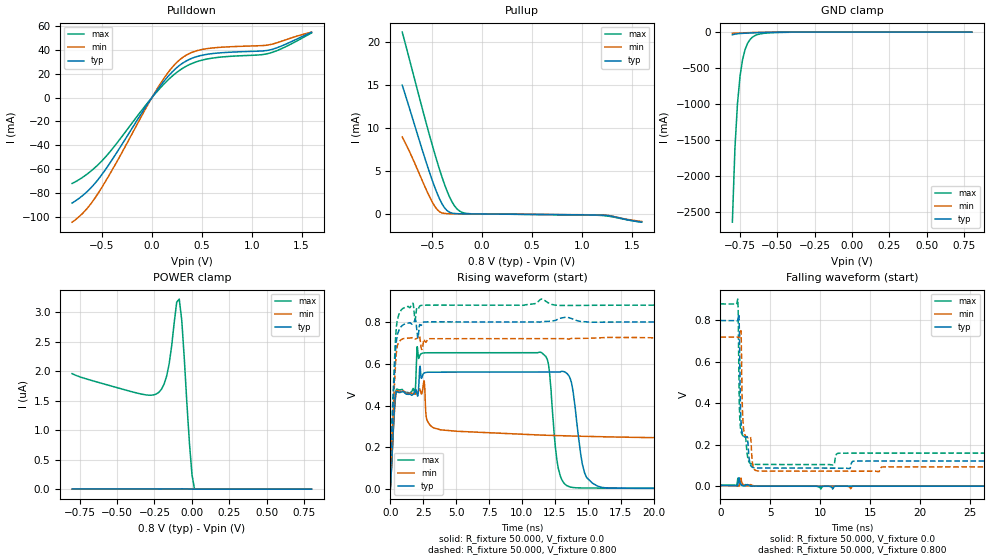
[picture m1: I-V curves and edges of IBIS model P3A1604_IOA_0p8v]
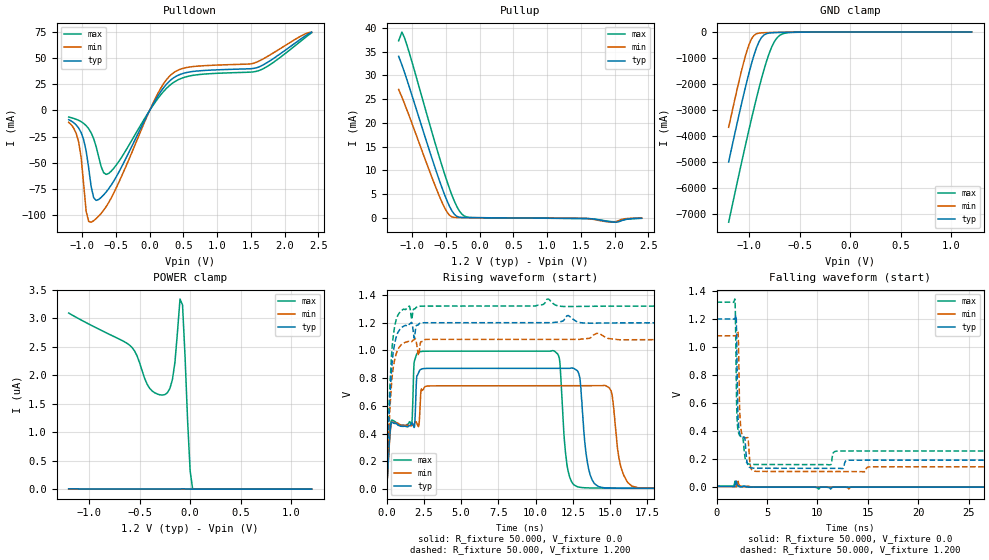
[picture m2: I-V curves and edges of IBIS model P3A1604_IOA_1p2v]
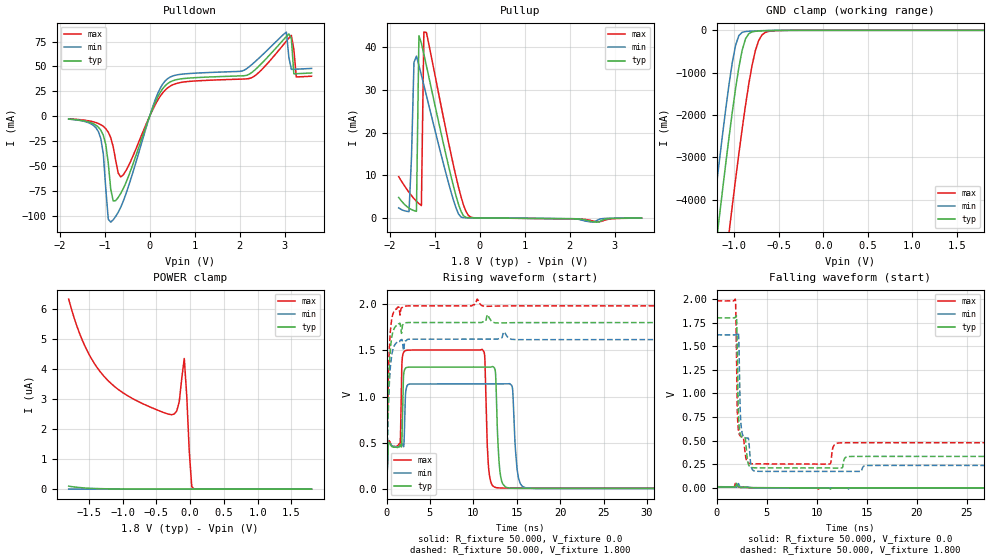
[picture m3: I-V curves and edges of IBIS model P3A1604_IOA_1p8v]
| NXP Semiconductors
| IBIS Model for P3A1604_WLCSP
| BIDIRECTIONAL VOLTAGE LEVEL TRANSLATOR WITH AUTO DIRECTION
| IBIS file created by T2B Version 21.1.4.11121.319246   004
| Cadence Design Systems, Inc. 2011
[IBIS ver] 5.0
[File name] p3a1604_wlcsp.ibs
[File Rev]  1.0
[Date]   July 30, 2024
[Source] NXP
[Notes]   The voltage level for A ports and B ports are
   different,for A side port, the voltage is 0.8v, 1.2V and 1.8V,
   for B side port, the voltage is 1.8v and 3.3V. In
   the model file, the model only contain the node voltage in
   the corresponding range.
   - Pin Description:
   - A1,B1,A2,B2,A3,B3,A4,B4 are the I/O pins.
   - VCCA Supply related to A pin
   - VCCB Supply related to B pin
   - OE is the Enable pin
   - All IO rising/falling waveforms has been verified on Cload=50pF in ADS.
   - IBIS SYNTAX CANNOT DESCRIBE THE CHARACTERISTICS OF
   ANY OUTPUT STRUCTURES THAT DYNAMICALLY CHANGES THE
   IMPEDANCES DURING THE TRANSITION. THIS DEVICE USES SIMILAR
   OUTPUT STRUCTURE AND THEREFORE THE SIMULATION RESULTS
   MAY NOT BE ACCURATE.
[Disclaimer]
NXP Semiconductors warrants and represents that the
IBIS model identified herein is owned by NXP Semiconductors.
The model provided is not warranted as fully representing
all of the operating characteristics and specifications of
the semiconductor products to which the model relates. Moreover,
unless there is a signed, written agreement to the contrary,
this IBIS model is furnished on an "as is" basis without
support or warranty of any kind, either expressed or implied,
regarding the use thereof, and NXP specifically disclaims
all implied warranties of merchantability and fitness of the
model for any purpose. NXP does not assume any liability arising
out of the application or use of this IBIS model including
infringement of patents and copyrights, nor does NXP convey
any license under its patents and copyrights or the rights of
others. NXP provides IBIS models as a service to our customers.
You and your company shall not distribute, convey, sell,
or give these models to anyone else without receiving prior
written permission from NXP Semiconductors.
NXP reserves the right to make changes
without notice to these IBIS models to improve reliability and gain.
This IBIS model is a property of NXP Semiconductors.
|   Component P3A1604
[Component] P3A1604
[Manufacturer] NXP
[Package]
| variable   typ   min   max
R_pkg   19.428m   5.881m   59.711m
L_pkg   1.154nH   1.074nH   1.308nH
C_pkg   0.159pF   0.155pF   0.163pF
[Pin]  signal_name   model_name   R_pin   L_pin   C_pin
B1   B1   P3A1604_IOB
VCCB   VCCB   Power
A1   A1   P3A1604_IOA
B2   B2   P3A1604_IOB
VCCA   VCCA   Power
A2   A2   P3A1604_IOA
B3   B3   P3A1604_IOB
OE   OE   P3A1604_OE
A3   A3   P3A1604_IOA
B4   B4   P3A1604_IOB
GND   GND   GND
A4   A4   P3A1604_IOA
| Model P3A1604_IOB
[Model Selector] 		P3A1604_IOB
P3A1604_IOB_1p8v 		1.8V VCCB supply
P3A1604_IOB_3p3v 		3.3V VCCB supply
| Model P3A1604_IOA
[Model Selector] 		P3A1604_IOA
P3A1604_IOA_0p8v   0.8V VCCA supply
P3A1604_IOA_1p2v 		1.2V VCCA supply
P3A1604_IOA_1p8v 		1.8V VCCA supply
| Model P3A1604_OE
[Model Selector] 		P3A1604_OE
P3A1604_OE_0p8v 		0.8V VCCA supply
P3A1604_OE_1p2v 		1.2V VCCA supply
P3A1604_OE_1p8v 		1.8V VCCA supply
| Models and submodels in the file (8): P3A1604_IOA_0p8v (I/O), P3A1604_IOA_1p2v (I/O), P3A1604_IOA_1p8v (I/O), P3A1604_OE_0p8v (Input), P3A1604_OE_1p2v (Input), P3A1604_OE_1p8v (Input), P3A1604_IOB_1p8v (I/O), P3A1604_IOB_3p3v (I/O)
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|   Model P3A1604_IOA_0p8v
[Model] P3A1604_IOA_0p8v
Model_type I/O
Polarity   Non-Inverting
Enable   Active-High
Vinl =  0.383V
Vinh =  0.407V
C_comp   6.7pF   6.3pF   7.44pF
[Model Spec]
Vinh   0.407V   0.327V   0.497V
Vinl   0.383V   0.309V   0.459V
[Temperature Range]   27.000   -40.000   125
[Voltage Range]   0.800V   0.720V   0.880V
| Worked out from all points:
|   slope of the pulldown table from 0 to 0.12 V, typ, clamps not added: 8.82 ohm
|   slope of the pullup table from 0 to 0.12 V, typ, clamps not added: 10 kohm
|   GND clamp passes 1 mA (typ) near -0.47 V on its own axis
|   rising waveform, R_fixture 50.000, V_fixture 0.800: 20-80 % time 291ps typ, 284ps min, 299ps max; typ from 0.12 V to 0.8 V
|   falling waveform, R_fixture 50.000, V_fixture 0.800: 20-80 % time 272ps typ, 940ps min, 160ps max; typ from 0.8 V to 0.121 V
[Pulldown]
|Voltage   I(typ)   I(min)   I(max)
-800mV    -88.25mA   -104.3mA   -71.84mA
-675mV    -80.6mA    -95.18mA   -65.59mA
-550mV    -69.67mA   -81.51mA   -57mA
-400mV    -52.1mA    -60.81mA   -43.27mA
50mV      5.924mA    7.002mA    4.898mA
175mV     19.01mA    22.42mA    15.82mA
300mV     28.37mA    33.08mA    24.1mA
400mV     32.87mA    37.8mA     28.51mA
550mV     36.19mA    40.96mA    32.25mA
1.175V    39.76mA    44.18mA    37.08mA
1.325V    44.11mA    47.88mA    41.96mA
1.6V      54.69mA    54.83mA    54.1mA
[Pullup]
|Voltage   I(typ)   I(min)   I(max)
-800mV    14.94mA    8.941mA    21.1mA
-725mV    12.16mA    7.184mA    17.8mA
-525mV    4.771mA    1.968mA    9.062mA
-475mV    3.131mA    912.8uA    7.025mA
-425mV    1.72mA     255uA      5.116mA
-375mV    697.9uA    59.31uA    3.394mA
-325mV    195.7uA    30.25uA    1.954mA
-275mV    56.06uA    23.59uA    919.1uA
-225mV    26.99uA    19.12uA    337.5uA
-100mV    10.03uA    8.488uA    19.31uA
1.2V      -132.1uA   -107.9uA   -175.7uA
1.6V      -936.5uA   -860.6uA   -952.5uA
[GND_clamp]
|Voltage   I(typ)   I(min)   I(max)
-800mV    -37.18mA   -17.65mA   -2.644A
-783mV    -28.7mA    -15.92mA   -1.621A
-766mV    -23.53mA   -14.29mA   -997.5mA
-749mV    -20.09mA   -12.72mA   -616.8mA
-732mV    -17.57mA   -11.23mA   -384.2mA
-715mV    -15.55mA   -9.817mA   -241.8mA
-698mV    -13.82mA   -8.483mA   -154.5mA
-681mV    -12.27mA   -7.234mA   -100.6mA
-664mV    -10.85mA   -6.076mA   -67.27mA
-596mV    -6.085mA   -2.462mA   -18.86mA
-460mV    -881.6uA   -140.2uA   -4.081mA
800mV     0A         0A         -554nA
[POWER_clamp]
|Voltage   I(typ)   I(min)   I(max)
-800mV    3.306nA    112.3pA    1.956uA
-339mV    2.632nA    68.92pA    1.611uA
-220mV    2.497nA    57.67pA    1.641uA
-169mV    2.57nA     53.78pA    1.908uA
-135mV    2.88nA     99.6pA     2.419uA
-101mV    3.887nA    100.7pA    3.167uA
-84mV     4.757nA    65.29pA    3.219uA
-67mV     5.276nA    47.8pA     2.852uA
-16mV     1.681nA    32.03pA    780.1nA
1mV       431.4pA    30.07pA    247.3nA
18mV      0A         28.45pA    0A
800mV     0A         0A         0A
[Ramp]
| variable   typ   min   max
dV/dt_r   0.476/0.338n   0.430/0.307n   0.523/0.368n
dV/dt_f   0.480/0.135n   0.432/0.157n   0.527/0.122n
R_load = 1.000M
[Rising Waveform]
R_fixture= 50.000
V_fixture= 0.0
V_fixture_min= 0.0
V_fixture_max= 0.0
|time   V(typ)   V(min)   V(max)
0s        133.1uV    69uV       159.1uV
450ps     463.2mV    463.2mV    474.4mV
1.87ns    468.6mV    454.6mV    455.5mV
2.05ns    449mV      458.7mV    681.4mV
11.48ns   559.7mV    258.6mV    653.3mV
12.86ns   559.9mV    255.9mV    74.22mV
14.16ns   321mV      253.6mV    6.509mV
16.62ns   4.885mV    250mV      5.212mV
51.01ns   3.976mV    2.665mV    5.156mV
200ns     3.976mV    3.042mV    5.156mV
[Rising Waveform]
R_fixture= 50.000
V_fixture= 0.800
V_fixture_min= 0.720
V_fixture_max= 0.880
|time   V(typ)   V(min)   V(max)
0s        120.5mV    92.54mV    158.4mV
390ps     649.1mV    587.2mV    710.5mV
520ps     731.5mV    681mV      802.2mV
1.72ns    792.6mV    724.8mV    888.9mV
1.88ns    810mV      718mV      808.3mV
2.09ns    722.8mV    726.4mV    864.6mV
2.39ns    787.2mV    667.6mV    879.3mV
2.56ns    799.2mV    716.6mV    879.9mV
11.5ns    801.2mV    720mV      909.1mV
200ns     800mV      720mV      880mV
[Falling Waveform]
R_fixture= 50.000
V_fixture= 0.0
V_fixture_min= 0.0
V_fixture_max= 0.0
|time   V(typ)   V(min)   V(max)
0s        3.937mV    3.009mV    5.156mV
1.59ns    2.873mV    3.109mV    2.966mV
1.69ns    1.42mV     2.754mV    20.53mV
1.75ns    9.832mV    1.733mV    39.14mV
1.86ns    41.07mV    173uV      19.05mV
2.05ns    9.896mV    39.47mV    6.138mV
2.21ns    4.046mV    11.27mV    2.695mV
2.67ns    7.654mV    1.294mV    5.15mV
11.22ns   -13.69mV   72.43uV    50.91uV
200ns     104.5nV    85.92nV    9.769uV
[Falling Waveform]
R_fixture= 50.000
V_fixture= 0.800
V_fixture_min= 0.720
V_fixture_max= 0.880
|time   V(typ)   V(min)   V(max)
0s        800mV      720mV      880mV
1.74ns    802.4mV    718.9mV    902.5mV
1.87ns    813.1mV    717.8mV    448.6mV
1.98ns    420.9mV    738.3mV    294.9mV
2.07ns    306.7mV    738.8mV    261.7mV
2.18ns    257.6mV    403.2mV    248.5mV
2.3ns     242.8mV    285.3mV    242.2mV
3.02ns    101.3mV    235.8mV    109.1mV
3.31ns    89.43mV    89.57mV    105.7mV
200ns     120.7mV    92.47mV    158.8mV
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|   Model P3A1604_IOA_1p2
[Model] P3A1604_IOA_1p2v
Model_type I/O
Polarity   Non-Inverting
Enable   Active-High
Vinl =  0.566V
Vinh =  0.616V
C_comp   6.7pF   6.3pF   7.44pF
[Model Spec]
Vinh   0.616V   0.506V   0.745V
Vinl   0.566V   0.475V   0.675V
[Temperature Range]   27.000   -40.000   125
[Voltage Range]   1.200V   1.080V   1.320V
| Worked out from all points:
|   slope of the pulldown table from 0 to 0.18 V, typ, clamps not added: 9.3 ohm
|   slope of the pullup table from 0 to 0.18 V, typ, clamps not added: 9.99 kohm
|   GND clamp passes 1 mA (typ) near -0.47 V on its own axis
|   rising waveform, R_fixture 50.000, V_fixture 1.200: 20-80 % time 355ps typ, 363ps min, 342ps max; typ from 0.19 V to 1.2 V
|   falling waveform, R_fixture 50.000, V_fixture 1.200: 20-80 % time 251ps typ, 940ps min, 155ps max; typ from 1.2 V to 0.191 V
[Pulldown]
|Voltage   I(typ)   I(min)   I(max)
-1.2V     -8.791mA   -11.31mA   -6.279mA
-1.052V   -16.73mA   -30.04mA   -9.411mA
-1.015V   -21.1mA    -44.92mA   -10.69mA
-941mV    -38.5mA    -96.13mA   -14.45mA
-867mV    -72.41mA   -106.4mA   -21.25mA
-793mV    -85.63mA   -103mA     -34.46mA
-682mV    -80.43mA   -95.02mA   -59.23mA
-608mV    -74.61mA   -87.76mA   -59.99mA
58mV      6.803mA    8.033mA    5.631mA
317mV     29.23mA    34mA       24.92mA
1.612V    41.26mA    46.78mA    37.82mA
2.4V      74.64mA    74.54mA    73.93mA
[Pullup]
|Voltage   I(typ)   I(min)   I(max)
-1.2V     34.02mA    27.03mA    37.32mA
-1.152V   32.22mA    25.42mA    39.14mA
-1.115V   30.7mA     24.1mA     37.98mA
-708mV    12.56mA    8.518mA    18.09mA
-523mV    4.978mA    2.212mA    9.373mA
-449mV    2.466mA    545.8uA    6.238mA
-375mV    714.3uA    59.81uA    3.495mA
-301mV    103.2uA    26.55uA    1.427mA
-227mV    27.61uA    19.4uA     356.3uA
1.549V    -157.4uA   -136.6uA   -185.8uA
1.993V    -941uA     -944.8uA   -847.4uA
2.4V      -100.4uA   -62.75uA   -130.4uA
[GND_clamp]
|Voltage   I(typ)   I(min)   I(max)
-1.2V     -4.983A    -3.655A    -7.298A
-1.05V    -2.369A    -1.134A    -4.614A
-1V       -1.581A    -489.3mA   -3.757A
-975mV    -1.218A    -263.8mA   -3.338A
-925mV    -597.9mA   -62.39mA   -2.53A
-875mV    -203.8mA   -28.3mA    -1.776A
-825mV    -58.48mA   -20.29mA   -1.107A
-775mV    -25.61mA   -15.08mA   -572.8mA
-700mV    -13.97mA   -8.614mA   -136.5mA
-625mV    -7.939mA   -3.793mA   -29.47mA
-500mV    -1.796mA   -351.8uA   -6.258mA
1.2V      0A         0A         -480.1nA
[POWER_clamp]
|Voltage   I(typ)   I(min)   I(max)
-1.2V     5.06nA     389.4pA    3.092uA
-600mV    3.501nA    116pA      2.531uA
-525mV    3.08nA     108.5pA    2.342uA
-400mV    2.86nA     96.72pA    1.771uA
-275mV    2.681nA    84.94pA    1.651uA
-175mV    2.688nA    76.82pA    1.925uA
-150mV    2.846nA    115.8pA    2.229uA
-100mV    4.196nA    118.7pA    3.337uA
-75mV     5.526nA    73.34pA    3.234uA
0V        600.1pA    49.12pA    321.1nA
25mV      0A         46.79pA    0A
1.2V      0A         0A         0A
[Ramp]
| variable   typ   min   max
dV/dt_r   0.714/1.848n   0.643/2.147n   0.785/1.658n
dV/dt_f   0.720/0.137n   0.648/0.162n   0.791/0.124n
R_load = 1.000M
[Rising Waveform]
R_fixture= 50.000
V_fixture= 0.0
V_fixture_min= 0.0
V_fixture_max= 0.0
|time   V(typ)   V(min)   V(max)
0s        46.24uV    63.83uV    153.5uV
340ps     481.3mV    480.9mV    497.7mV
1.68ns    476.1mV    458.5mV    462.2mV
2.12ns    831.9mV    453.3mV    986.1mV
11.14ns   871.1mV    745.6mV    999mV
11.63ns   871.1mV    745.6mV    910.1mV
12.17ns   870.8mV    745.6mV    133mV
13.29ns   344.8mV    745.6mV    10.05mV
16.91ns   6.053mV    8.967mV    7.731mV
200ns     5.974mV    4.591mV    7.721mV
[Rising Waveform]
R_fixture= 50.000
V_fixture= 1.200
V_fixture_min= 1.080
V_fixture_max= 1.320
|time   V(typ)   V(min)   V(max)
0s        190.3mV    144mV      254.5mV
400ps     940.3mV    838.8mV    1.056V
980ps     1.162V     1.04V      1.286V
1.53ns    1.19V      1.064V     1.32V
1.69ns    1.201V     1.063V     1.223V
1.93ns    1.145V     1.084V     1.302V
2.17ns    1.191V     964.1mV    1.318V
2.66ns    1.2V       1.08V      1.32V
10.78ns   1.2V       1.08V      1.371V
200ns     1.2V       1.08V      1.32V
[Falling Waveform]
R_fixture= 50.000
V_fixture= 0.0
V_fixture_min= 0.0
V_fixture_max= 0.0
|time   V(typ)   V(min)   V(max)
0s        5.974mV    4.591mV    7.721mV
1.67ns    5.096mV    4.627mV    5.787mV
1.77ns    3.793mV    4.35mV     22.7mV
1.84ns    13.47mV    3.376mV    42.61mV
1.94ns    43.92mV    2.385mV    20.42mV
2.14ns    10.38mV    42.01mV    7.134mV
2.29ns    4.836mV    11.93mV    3.931mV
2.84ns    6.943mV    1.693mV    3.728mV
11.31ns   -13.75mV   71.75uV    45.43uV
200ns     106.3nV    86.99nV    11.02uV
[Falling Waveform]
R_fixture= 50.000
V_fixture= 1.200
V_fixture_min= 1.080
V_fixture_max= 1.320
|time   V(typ)   V(min)   V(max)
0s        1.2V       1.08V      1.32V
1.82ns    1.203V     1.079V     1.342V
1.88ns    1.217V     1.078V     1.203V
1.96ns    1.198V     1.079V     702.8mV
2.09ns    582.7mV    1.104V     431.2mV
2.17ns    451.2mV    1.053V     392.1mV
2.39ns    366.3mV    433.6mV    362mV
3.11ns    156.4mV    351.7mV    167.7mV
3.37ns    138.2mV    147.4mV    163mV
200ns     191mV      144.1mV    256.1mV
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|   Model P3A1604_IOA_1p8
[Model] P3A1604_IOA_1p8v
Model_type I/O
Polarity   Non-Inverting
Enable   Active-High
Vinl =  0.857V
Vinh =  0.954V
C_comp   6.7pF   6.3pF   7.44pF
[Model Spec]
Vinh   0.954V   0.786V   1.148V
Vinl   0.857V   0.710V   1.031V
[Temperature Range]   27.000   -40.000   125
[Voltage Range]   1.800V   1.620V   1.980V
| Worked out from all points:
|   slope of the pulldown table from 0 to 0.27 V, typ, clamps not added: 10.2 ohm
|   slope of the pullup table from 0 to 0.27 V, typ, clamps not added: 9.99 kohm
|   GND clamp passes 1 mA (typ) near -0.46 V on its own axis
|   rising waveform, R_fixture 50.000, V_fixture 1.800: 20-80 % time 328ps typ, 356ps min, 306ps max; typ from 0.324 V to 1.8 V
|   falling waveform, R_fixture 50.000, V_fixture 1.800: 20-80 % time 212ps typ, 929ps min, 132ps max; typ from 1.8 V to 0.327 V
[Pulldown]
|Voltage   I(typ)   I(min)   I(max)
-1.8V     -2.844mA   -2.935mA   -2.583mA
-1.14V    -10.96mA   -15.4mA    -7.275mA
-975mV    -28.51mA   -72.7mA    -12.47mA
-865mV    -73.24mA   -106.4mA   -21.51mA
-590mV    -73mA      -85.73mA   -59.07mA
400mV     32.81mA    37.73mA    28.46mA
2.16V     41.14mA    47.9mA     37.54mA
3.04V     80.08mA    84.49mA    75.46mA
3.15V     78mA       47.06mA    81.26mA
3.205V    42.61mA    47.16mA    67.3mA
3.26V     42.71mA    47.26mA    39.46mA
3.6V      43.47mA    48.03mA    40.18mA
[Pullup]
|Voltage   I(typ)   I(min)   I(max)
-1.8V     4.797mA    2.358mA    9.687mA
-1.57V    2.288mA    1.45mA     5.987mA
-1.515V   1.956mA    14.21mA    5.228mA
-1.46V    1.715mA    36.48mA    4.53mA
-1.405V   1.54mA     37.96mA    3.902mA
-1.35V    42.75mA    35.79mA    3.351mA
-1.295V   40.98mA    33.49mA    2.885mA
-1.24V    38.43mA    31.15mA    43.6mA
-1.185V   35.78mA    28.79mA    43.54mA
-525mV    5.164mA    2.325mA    9.649mA
-250mV    36.65uA    21.43uA    587.6uA
3.6V      -33.88uA   -21.05uA   -51.13uA
[GND_clamp]
|Voltage   I(typ)   I(min)   I(max)
-1.8V     -16.37A    -15.08A    -18.65A
-1.282V   -6.486A    -5.156A    -8.809A
-1.245V   -5.804A    -4.473A    -8.124A
-1.171V   -4.46A     -3.137A    -6.77A
-1.06V    -2.534A    -1.283A    -4.789A
-1.023V   -1.935A    -761mA     -4.148A
-986mV    -1.374A    -352.6mA   -3.521A
-912mV    -469.7mA   -46.7mA    -2.328A
-838mV    -79.3mA    -21.9mA    -1.27A
-764mV    -22.84mA   -14.06mA   -479.8mA
-653mV    -9.989mA   -5.387mA   -50mA
1.8V      0A         0A         -450.9nA
[POWER_clamp]
|Voltage   I(typ)   I(min)   I(max)
-1.8V     100nA      2.938nA    6.343uA
-1.641V   54.74nA    1.584nA    5.211uA
-1.419V   23.49nA    802.9pA    4.194uA
-790mV    5.021nA    397pA      2.948uA
-235mV    3.606nA    271.7pA    2.508uA
-161mV    3.723nA    214.6pA    2.921uA
-87mV     6.18nA     119pA      4.36uA
-50mV     6.217nA    87.03pA    3.105uA
-13mV     2.171nA    79.13pA    1.261uA
24mV      0A         75.36pA    87.55nA
61mV      0A         72.31pA    0A
1.8V      0A         0A         0A
[Ramp]
| variable   typ   min   max
dV/dt_r   1.071/1.745n   0.964/2.007n   1.177/1.572n
dV/dt_f   1.080/0.141n   0.972/0.166n   1.185/0.127n
R_load = 1.000M
[Rising Waveform]
R_fixture= 50.000
V_fixture= 0.0
V_fixture_min= 0.0
V_fixture_max= 0.0
|time   V(typ)   V(min)   V(max)
0s        426.6uV    366.9uV    367.4uV
1.56ns    482.9mV    464.7mV    482.2mV
1.99ns    1.251V     470.3mV    1.482V
2.48ns    1.318V     1.13V      1.502V
10.99ns   1.319V     1.137V     1.51V
11.81ns   1.319V     1.137V     182.5mV
12.84ns   486.5mV    1.137V     14.57mV
14.5ns    10.52mV    1.096V     11.66mV
16.05ns   9.039mV    13.81mV    11.59mV
200ns     8.966mV    6.891mV    11.57mV
[Rising Waveform]
R_fixture= 50.000
V_fixture= 1.800
V_fixture_min= 1.620
V_fixture_max= 1.980
|time   V(typ)   V(min)   V(max)
0s        324mV      232.3mV    462.9mV
70ps      482.4mV    391.2mV    616.5mV
250ps     1.145V     970.4mV    1.333V
370ps     1.41V      1.224V     1.61V
590ps     1.635V     1.441V     1.831V
890ps     1.738V     1.55V      1.926V
10.43ns   1.8V       1.62V      2.054V
11.61ns   1.884V     1.62V      1.975V
12.78ns   1.795V     1.622V     1.978V
200ns     1.8V       1.62V      1.98V
[Falling Waveform]
R_fixture= 50.000
V_fixture= 0.0
V_fixture_min= 0.0
V_fixture_max= 0.0
|time   V(typ)   V(min)   V(max)
0s        8.966mV    6.891mV    11.57mV
1.81ns    7.778mV    6.768mV    21.79mV
1.89ns    16.8mV     5.893mV    46.65mV
2ns       47.06mV    6.188mV    21.69mV
2.19ns    12.81mV    44.66mV    7.605mV
2.29ns    7.439mV    18.61mV    4.632mV
2.51ns    2.681mV    7.098mV    4.983mV
10.18ns   77.34uV    117.8uV    -14.43mV
11.36ns   -13.81mV   84.43uV    44.23uV
200ns     113.3nV    86.97nV    13.72uV
[Falling Waveform]
R_fixture= 50.000
V_fixture= 1.800
V_fixture_min= 1.620
V_fixture_max= 1.980
|time   V(typ)   V(min)   V(max)
0s        1.8V       1.62V      1.98V
1.87ns    1.805V     1.619V     1.997V
1.94ns    1.818V     1.619V     1.79V
2.02ns    1.76V      1.622V     1.141V
2.17ns    832mV      1.645V     626.1mV
2.47ns    542.7mV    636.8mV    539.7mV
3.51ns    214.4mV    208.9mV    254.5mV
11.23ns   210.2mV    173mV      251mV
12.63ns   246.7mV    173mV      476.9mV
200ns     327.3mV    233.4mV    469.9mV
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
